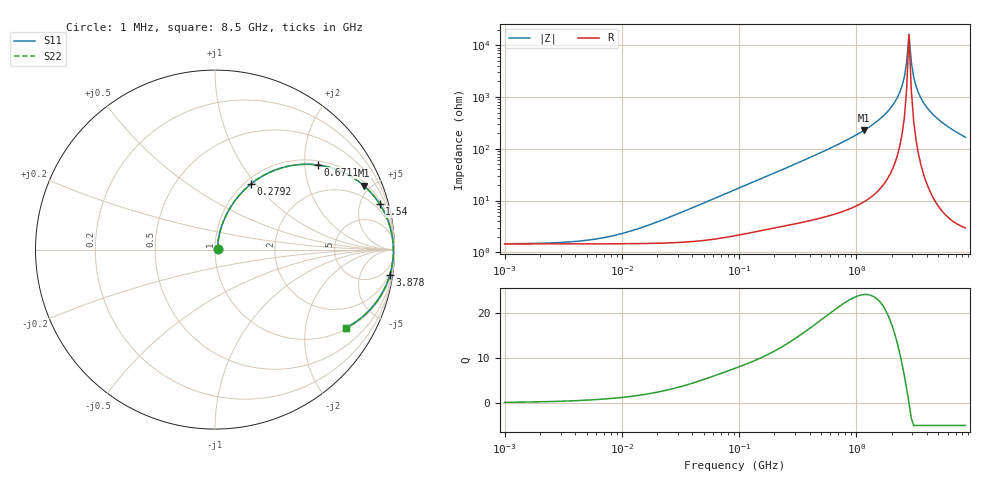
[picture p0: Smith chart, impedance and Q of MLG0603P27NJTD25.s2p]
! S-Parameter Data Generated by TDK Corporation
! Copyright(C) 2025 TDK Corporation.
! All Rights Reserved.
! TDK P/N: MLG0603P27NJTD25 (SMD / SMT Inductor (Coil))
! Property: L=27nH at 500MHz
! Size(LxWxT): 0.6x0.3x0.3mm
! Model Type: s2p (Touchstone File Format Version 1.0)
! Frequency: DC=Yes Start=1MHz Stop=8500MHz 198points Log-sweep
! Model Generated on Feb. 6, 2025
! Terms and conditions regarding TDK Simulation Models:
! 1)This simulation model is being provided solely for informational
!  purposes. Please refer to the specifications of the products in
!  terms of detailed characteristics of such products.
! 2)In no event shall TDK Corporation of any of its subsidiaries be
!  liable for any loss or damage arising, directly or indirectly,
!  from any information contained in this simulation model, including,
!  but not limited to loss or damages arising from any inaccuracies,
!  omissions or errors in connection with such information.
! 3)Any and all copyrights on this simulation model are owned by
!  TDK Corporation.  Duplication or redistribution of this simulation
!  model without prior written permission from TDK Corporation
!  is prohibited.
! 4)This simulation model is subject to any modification or change
!  without any prior notice.
! 5)Neither TDK Corporation nor any of its subsidiaries shall make any
!  warranty, express or implied, including but not limited to the
!  correctness, implied warranties of merchantability and fitness for
!  a particular purpose with respect to this simulation models.
! 6)The use of this simulation model shall be deemed to have consented
!  to the terms and conditions hereof.
! Port Assignments:
!  1 ---@@@--- 2
! Applicable Conditions:
!  Temperature = 25 degC
!  DC Bias Current = 0 A
!  Small Signal Operation
# Hz S MA R 50
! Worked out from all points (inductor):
!   197 points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, 1 MHz to 8.5 GHz, reference 50 ohm
!   read as one part in series: L = 28.2 nH near 26.51 MHz
!   highest Q = 24 at 1.168 GHz (marker M1), where L = 31.1 nH
!   self-resonance near 2.807 GHz
!   S11 on the Smith chart (normalised r, x): 1 MHz: 1.03, +0.00; 279.2 MHz: 1.07, +0.94; 671.1 MHz: 1.11, +2.32; 1.54 GHz: 1.31, +7.11; 3.878 GHz: 2, -14; 8.5 GHz: 1.06, -3.34
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1000000  0.0144 6.9  0.9857 -0.1  0.9857 -0.1  0.0144 6.9
4587603  0.01642 28.9  0.9857 -0.5  0.9857 -0.5  0.01642 28.9
9601846  0.02215 48.5  0.9855 -1.0  0.9855 -1.0  0.02215 48.5
2.10461e7  0.03967 66.1  0.9846 -2.1  0.9846 -2.1  0.03967 66.1
9.219544e7  0.1563 73.7  0.9677 -8.9  0.9677 -8.9  0.1563 73.7
1.680096e8  0.2694 69.0  0.9378 -15.6  0.9378 -15.6  0.2694 69.0
2.791662e8  0.4148 61.4  0.8803 -24.4  0.8803 -24.4  0.4148 61.4
4.229561e8  0.566 52.2  0.7918 -34.4  0.7918 -34.4  0.566 52.2
6.710824e8  0.7411 39.5  0.6369 -47.8  0.6369 -47.8  0.7411 39.5
1.167757e9  0.9026 23.2  0.3946 -64.4  0.3946 -64.4  0.9026 23.2
1.540426e9  0.9519 15.5  0.2676 -72.0  0.2676 -72.0  0.9519 15.5
1.940355e9  0.9777 9.4  0.1636 -77.5  0.1636 -77.5  0.9777 9.4
2.333852e9  0.9894 4.7  0.08178 -80.2  0.08178 -80.2  0.9894 4.7
2.559585e9  0.9925 2.3  0.04134 -78.4  0.04134 -78.4  0.9925 2.3
2.680511e9  0.9934 1.2  0.02146 -71.5  0.02146 -71.5  0.9934 1.2
2.80715e9  0.9939 0.0  0.006151 -1.6  0.006151 -1.6  0.9939 0.0
2.939772e9  0.9939 -1.2  0.02102 72.4  0.02102 72.4  0.9939 -1.2
3.07866e9  0.9934 -2.3  0.04094 79.6  0.04094 79.6  0.9934 -2.3
3.37643e9  0.9912 -4.7  0.08163 81.5  0.08163 81.5  0.9912 -4.7
3.877948e9  0.9844 -8.2  0.1435 79.7  0.1435 79.7  0.9844 -8.2
5.357206e9  0.9507 -17.0  0.2922 71.9  0.2922 71.9  0.9507 -17.0
8.5e9  0.851 -30.7  0.5103 58.3  0.5103 58.3  0.851 -30.7
